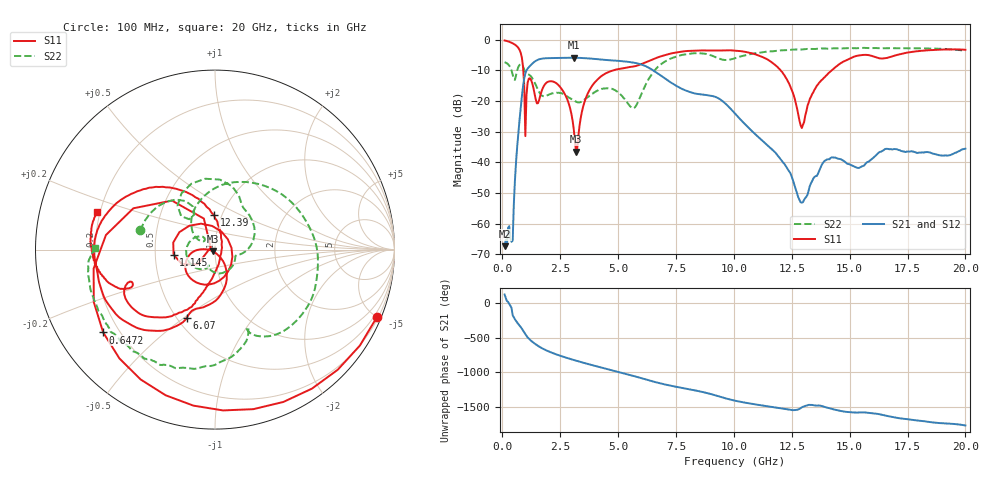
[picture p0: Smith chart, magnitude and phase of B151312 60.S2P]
!  2-Port S-parameters saved by WinCal
! VAR MeasName=S-Parameters (CALIBRATED_DATA) read from VNA (N5244A)
! VAR MeasDate=12/8/2015 5:48:28 PM
! VAR NAME=B151312 60
! VAR FILENAME=B151312 60.S2P
! VAR DATE=12/8/2015 5:48:28 PM
! VAR PHYS_PORTS=1,2
# Hz S DB R 50
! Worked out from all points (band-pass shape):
!   401 points, 100 MHz to 20 GHz, reference 50 ohm
!   highest |S21| = -5.84 dB at 3.085 GHz (marker M1); lowest = -67.4 dB at 100 MHz (marker M2)
!   |S21| within 3 dB of the highest: 1.157 GHz to 6.258 GHz (5.101 GHz wide, 138 % of centre)
!   lowest |S11| = -36.6 dB at 3.184 GHz (marker M3), VSWR 1.03, Z = 48.9 - j0.979 ohm
!   |S11| at or under -10 dB: 906.1 MHz to 4.771 GHz (3.865 GHz wide, 136 % of centre); 12.02 GHz to 14.22 GHz (2.195 GHz wide, 16.7 % of centre)
!   |S22| runs from -22.3 to -2.6 dB; largest |S21 - S12| = 0.0017
!   S11 on the Smith chart (normalised r, x): 100 MHz: 0.30, -4.99; 647.2 MHz: 0.14, -0.32; 1.145 GHz: 0.62, -0.04; 6.07 GHz: 0.56, -0.51; 12.39 GHz: 0.92, +0.37; 20 GHz: 0.19, +0.15
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1e8  -0.20 -22.6  -67.40 126.8  -67.49 135.0  -7.33 165.6
3.985e8  -0.94 -87.2  -65.99 -66.2  -64.14 -60.1  -10.01 121.2
6.4725e8  -2.21 -143.5  -34.52 80.4  -34.56 80.2  -9.85 130.4
8.4625e8  -5.85 153.2  -18.44 -6.1  -18.44 -6.2  -8.16 86.1
9.955e8  -31.44 153.6  -10.98 -86.4  -10.99 -86.4  -10.51 60.7
1.14475e9  -12.67 -173.0  -8.94 -150.6  -8.94 -150.6  -11.35 44.7
1.692e9  -16.93 -59.4  -6.17 74.6  -6.17 74.6  -18.12 -14.7
2.23925e9  -13.75 -139.7  -5.94 -7.5  -5.94 -7.5  -17.33 -51.6
3.085e9  -29.08 -179.0  -5.84 -99.7  -5.84 -99.7  -19.73 -110.3
3.1845e9  -36.57 -137.6  -5.85 -109.5  -5.86 -109.5  -20.19 -110.9
3.43325e9  -23.69 -55.1  -5.93 -133.3  -5.92 -133.3  -20.15 -112.4
4.876e9  -9.75 -100.8  -6.79 100.3  -6.79 100.2  -16.45 165.1
6.07e9  -7.73 -112.5  -8.22 -9.0  -8.21 -9.1  -16.67 143.9
6.7665e9  -5.58 -121.4  -11.24 -73.1  -11.22 -73.2  -8.51 79.3
7.861e9  -3.73 -143.9  -16.36 -150.1  -16.35 -150.5  -4.81 -4.6
1.005e10  -3.49 173.2  -24.06 31.5  -24.04 31.0  -6.00 -68.3
1.238825e10  -14.32 91.8  -42.93 -96.5  -43.00 -96.2  -3.33 -105.1
1.29355e10  -28.80 -6.3  -53.18 -64.1  -53.43 -65.5  -3.14 -112.7
1.338325e10  -17.68 -90.9  -46.10 -30.5  -46.16 -30.6  -2.99 -117.5
1.4826e10  -6.77 -125.2  -40.01 -129.3  -40.04 -129.4  -2.74 -134.4
1.67165e10  -5.70 -155.8  -35.73 164.1  -35.61 163.7  -2.69 -152.0
2e10  -3.24 162.1  -35.55 33.3  -35.72 32.7  -3.51 179.2
